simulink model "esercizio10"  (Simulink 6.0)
settings: Solver=ode45  StartTime=0.0  StopTime=5.0  RelTol=1e-3
undefined symbols (not defined in the file or in its folder): k
libraries: simulink x1

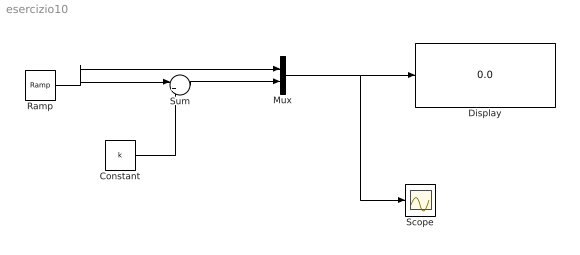
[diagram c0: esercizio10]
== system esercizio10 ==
  Constant : Constant  Value=k
  Display : Display
  Mux : Mux  Inputs=2
  Ramp : simulink/Sources/Ramp  slope=5  start=0  X0=0
  Scope : Scope
  Sum : Sum  Inputs=|++
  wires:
  Ramp/1 -> Sum/1, Mux/1
  Constant/1 -> Sum/2
  Sum/1 -> Mux/2
  Mux/1 -> Display/1, Scope/1
